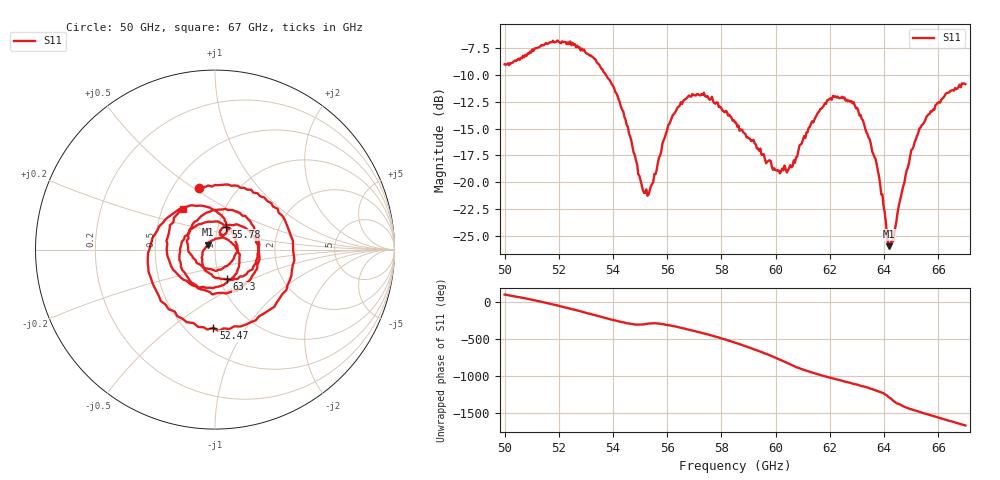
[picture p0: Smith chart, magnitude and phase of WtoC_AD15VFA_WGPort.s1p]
!Agilent Technologies,E8361A,US42410132,A.06.03.05
!Agilent E8361A: A.06.03.05
!Date: Friday, July 11, 2008 15:50:01
!Correction: S11(Full 2 Port(1,2))
!S1P File: Measurement: S11:
# Hz S  MA  R 50
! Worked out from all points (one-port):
!   401 points, 50 GHz to 67 GHz, reference 50 ohm
!   lowest |S11| = -26.0 dB at 64.19 GHz (marker M1), VSWR 1.11, Z = 45.9 + j2.58 ohm
!   |S11| at or under -10 dB: 53.74 GHz to end of sweep
!   S11 on the Smith chart (normalised r, x): 50 GHz: 0.67, +0.53; 52.47 GHz: 0.67, -0.72; 55.78 GHz: 1.09, +0.28; 63.3 GHz: 1.08, -0.37; 67 GHz: 0.64, +0.31
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5e10  0.3554 104.5
5.068e10  0.3897 58.9
5.13175e10  0.4304 9.6
5.17425e10  0.4501 -26.0
5.2125e10  0.4544 -60.0
5.2465e10  0.4364 -91.2
5.32725e10  0.3823 -168.8
5.37825e10  0.3096 140.8
5.425e10  0.2364 97.4
5.5185e10  0.08922 64.5
5.578e10  0.1395 65.1
5.6375e10  0.2229 24.9
5.69275e10  0.2581 -24.5
5.7565e10  0.2426 -83.5
5.85e10  0.1898 170.9
5.9095e10  0.1556 96.1
5.97325e10  0.1259 8.8
6.0625e10  0.1186 -136.2
6.1135e10  0.1705 151.9
6.173e10  0.2239 84.3
6.275e10  0.2378 -14.5
6.33025e10  0.1782 -67.9
6.4195e10  0.05028 146.2
6.4875e10  0.1167 3.2
6.53e10  0.1779 -47.1
6.5895e10  0.2288 -112.4
6.64475e10  0.2669 -171.7
6.7e10  0.2871 128.6
